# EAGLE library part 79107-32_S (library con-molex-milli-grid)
RECEPTACAL
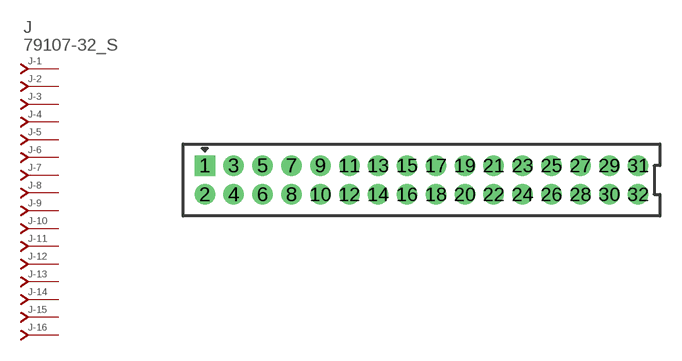
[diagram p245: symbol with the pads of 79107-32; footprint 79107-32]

Designator prefix J; gates -1=J-NV -2=J-N -3=J-N -4=J-N -5=J-N -6=J-N -7=J-N -8=J-N -9=J-N -10=J-N -11=J-N -12=J-N -13=J-N -14=J-N -15=J-N -16=J-N -17=J-N -18=J-N -19=J-N -20=J-N -21=J-N -22=J-N -23=J-N -24=J-N -25=J-N -26=J-N -27=J-N -28=J-N -29=J-N -30=J-N -31=J-N -32=J-N

## 79107-32_S  [79107-32]
1  -1:J  pas
2  -2:J  pas
3  -3:J  pas
4  -4:J  pas
5  -5:J  pas
6  -6:J  pas
7  -7:J  pas
8  -8:J  pas
9  -9:J  pas
10  -10:J  pas
11  -11:J  pas
12  -12:J  pas
13  -13:J  pas
14  -14:J  pas
15  -15:J  pas
16  -16:J  pas
17  -17:J  pas
18  -18:J  pas
19  -19:J  pas
20  -20:J  pas
21  -21:J  pas
22  -22:J  pas
23  -23:J  pas
24  -24:J  pas
25  -25:J  pas
26  -26:J  pas
27  -27:J  pas
28  -28:J  pas
29  -29:J  pas
30  -30:J  pas
31  -31:J  pas
32  -32:J  pas

## Footprint 79107-32 (pad centres in mm)
RECEPTACAL Dual Row, Vertical, Through-Hole
drill 0.914 square: 1 -15,1
drill 0.914: 2 -15,-1; 3 -13,1; 4 -13,-1; 5 -11,1; 6 -11,-1; 7 -9,1; 8 -9,-1; 9 -7,1; 10 -7,-1; 11 -5,1; 12 -5,-1; 13 -3,1; 14 -3,-1; 15 -1,1; 16 -1,-1; 17 1,1; 18 1,-1; 19 3,1; 20 3,-1; 21 5,1; 22 5,-1; 23 7,1; 24 7,-1; 25 9,1; 26 9,-1; 27 11,1; 28 11,-1; 29 13,1; 30 13,-1; 31 15,1; 32 15,-1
